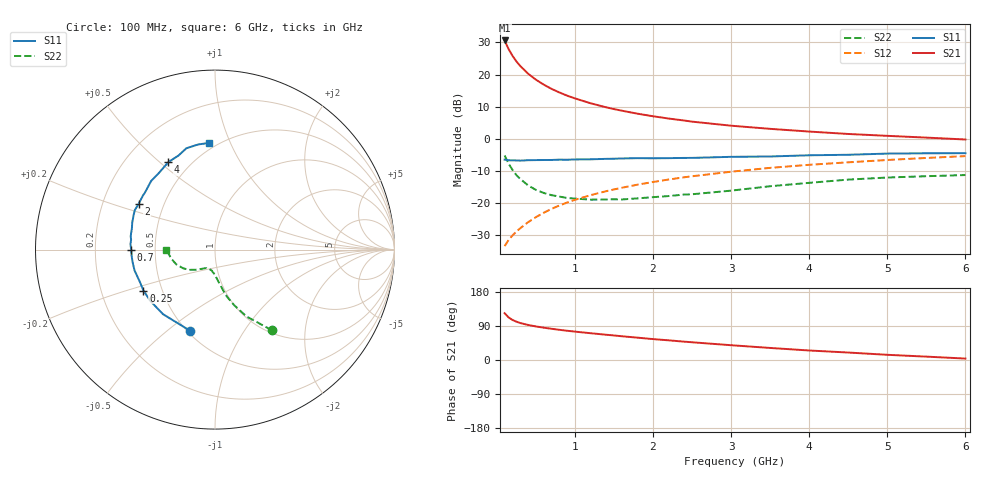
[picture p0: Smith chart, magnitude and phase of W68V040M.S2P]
! SIEMENS Small Signal Semiconductors
! BFR193W
! Si NPN RF Bipolar Junction Transistor in SOT323
! VCE = 8 V  IC = 40 mA
! Common Emitter S-Parameters:  September  1992
# GHz  S  MA  R  50
!  f  S11  S21  S12  S22
! GHz  MAG  ANG  MAG  ANG  MAG  ANG  MAG  ANG
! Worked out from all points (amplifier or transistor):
!   28 points, 100 MHz to 6 GHz, reference 50 ohm
!   highest |S21| = 30.6 dB at 100 MHz (marker M1)
!   |S21| within 3 dB of that: start of sweep to 158.8 MHz
!   unconditionally stable (mu >= 1): 622.9 MHz to 2.647 GHz
!   at 300 MHz: K = 0.87, MSG = 25.3 dB, |S12| = -27.9 dB
!   at 1.5 GHz: K = 1.03, MAG = 11.4 dB, |S12| = -15.8 dB
!   at 6 GHz: K = 0.92, MSG = 2.6 dB, |S12| = -5.4 dB
!   S11 on the Smith chart (normalised r, x): 100 MHz: 0.52, -0.60; 250 MHz: 0.39, -0.23; 700 MHz: 0.36, -0.00; 2 GHz: 0.36, +0.24; 4 GHz: 0.38, +0.53; 6 GHz: 0.46, +0.84
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0.1  0.4724 -107.4  33.94 123.5  0.0212 59.3  0.5499 -54.8
0.15  0.4619 -128.9  25.07 112.6  0.0264 59.5  0.4114 -64.8
0.2  0.4599 -141.6  19.65 105.7  0.031 61.1  0.3286 -70.9
0.25  0.4594 -150.2  16.07 101.2  0.0358 62.9  0.272 -75.6
0.3  0.4556 -156.5  13.59 97.6  0.0403 64.8  0.2365 -78.3
0.4  0.4629 -165.4  10.32 92.5  0.05 67.4  0.1877 -82.9
0.5  0.4645 -171.3  8.323 88.6  0.0599 69.0  0.1598 -86.5
0.6  0.4659 -176.1  6.975 85.3  0.0702 70.0  0.1431 -90.4
0.7  0.4668 -179.8  5.982 82.4  0.0807 70.5  0.1321 -92.8
0.8  0.472 176.4  5.267 79.7  0.091 70.7  0.1258 -95.9
0.9  0.4705 173.4  4.687 77.2  0.1014 70.7  0.1193 -98.1
1  0.4758 170.9  4.253 74.9  0.1116 70.5  0.1169 -100.3
1.2  0.4779 165.7  3.569 70.7  0.1321 69.9  0.1125 -106.2
1.5  0.488 159.5  2.897 64.7  0.1621 68.3  0.1139 -112.9
2  0.4957 149.2  2.239 55.2  0.2119 65.0  0.1229 -121.4
2.2  0.4983 146.0  2.063 51.9  0.2314 63.4  0.1279 -123.6
3  0.5223 132.9  1.596 39.0  0.3065 56.9  0.1554 -133.7
3.5  0.5288 126.4  1.425 31.8  0.3517 52.7  0.182 -141.7
4  0.5522 118.1  1.293 25.1  0.3925 48.3  0.2055 -149.5
4.5  0.5624 111.1  1.186 19.7  0.4291 44.2  0.2308 -159.1
5.5  0.5933 99.1  1.041 8.9  0.5016 36.1  0.2607 -175.4
6  0.5952 93.1  0.973 3.8  0.5358 31.8  0.2718 -179.8
